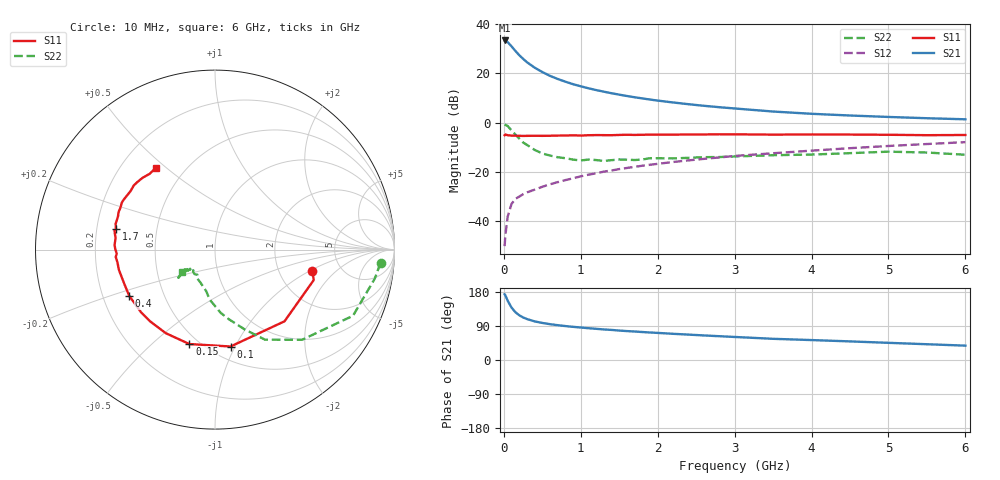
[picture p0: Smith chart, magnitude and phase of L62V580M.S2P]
!  INFINEON TECHNOLOGIES Small Signal Semiconductors
! BFR380L3 , Si-NPN RF-Transistor in TSLP-3-1
!  Vce=2.5 V,  Ic=80 mA
! Common Emitter S-Parameters:  07. March 2005
#  GHz  S  MA  R  50
! f  S11  S21  S12  S22
! GHz  Mag  Ang  Mag  Ang  Mag  Ang  Mag  Ang
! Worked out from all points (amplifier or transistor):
!   36 points, 10 MHz to 6 GHz, reference 50 ohm
!   highest |S21| = 33.4 dB at 10 MHz (marker M1)
!   |S21| within 3 dB of that: start of sweep to 116.4 MHz
!   unconditionally stable (mu >= 1): 1.116 GHz to 4.933 GHz
!   at 250 MHz: K = 0.57, MSG = 27.5 dB, |S12| = -29.1 dB
!   at 1.4 GHz: K = 1.03, MAG = 14.6 dB, |S12| = -19.4 dB
!   at 6 GHz: K = 0.98, MSG = 4.6 dB, |S12| = -7.9 dB
!   S11 on the Smith chart (normalised r, x): 10 MHz: 3.09, -1.08; 100 MHz: 0.62, -0.96; 150 MHz: 0.44, -0.66; 400 MHz: 0.31, -0.23; 1.7 GHz: 0.28, +0.10; 6 GHz: 0.35, +0.46
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0.01  0.5562 -12.5  46.84 173.5  0.0031 76.2  0.9253 -4.6
0.02  0.5758 -17.1  46.56 170.5  0.0052 78.9  0.9048 -10.3
0.05  0.5564 -45.9  43.19 156.3  0.0124 69.9  0.8527 -25.6
0.1  0.5468 -80.9  35.55 138.4  0.0224 61.0  0.6984 -46.0
0.15  0.5452 -105.2  28.73 126.1  0.0283 54.2  0.5746 -60.9
0.2  0.5405 -120.5  23.56 118.1  0.0315 53.9  0.4755 -69.5
0.25  0.5388 -131.9  19.84 112.4  0.0352 52.5  0.3972 -78.5
0.3  0.54 -139.8  16.95 108.1  0.0383 54.1  0.3542 -84.8
0.4  0.543 -151.6  13.14 101.9  0.0436 55.5  0.2802 -96.0
0.5  0.5402 -159.2  10.7 97.8  0.0498 58.0  0.237 -101.9
0.6  0.5429 -164.6  8.939 94.5  0.056 60.1  0.2152 -108.2
0.7  0.5473 -168.2  7.737 91.9  0.062 61.8  0.1987 -114.8
0.9  0.5547 -175.8  6.049 87.5  0.0742 64.3  0.1778 -124.9
1.1  0.5559 179.6  5.002 83.9  0.0878 65.6  0.1779 -129.4
1.4  0.5573 173.5  3.968 79.4  0.1069 67.0  0.1733 -135.1
1.7  0.564 168.1  3.288 75.2  0.127 67.5  0.1743 -142.3
2.2  0.5713 161.1  2.574 69.1  0.159 67.7  0.1884 -142.3
2.8  0.5813 153.2  2.064 62.8  0.1966 67.3  0.2003 -147.0
3.5  0.5723 145.2  1.685 55.9  0.2395 64.8  0.2186 -144.7
4.5  0.5737 139.1  1.399 49.1  0.3035 62.8  0.2404 -143.4
5.5  0.5575 130.8  1.232 41.6  0.3687 58.7  0.2476 -143.0
6  0.5623 125.8  1.172 37.9  0.4023 56.4  0.2233 -145.8
